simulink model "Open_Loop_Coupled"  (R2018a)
settings: Solver=ode45  StartTime=0.0  StopTime=80  RelTol=1e-3  EnableMultiTasking=on
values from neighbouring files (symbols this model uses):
  Aact = [0, 1; -omg^2, -2*zet*omg]    [init.m]
  Bact = [0; omg^2]    [init.m]
  Cact = [1, 0]    [init.m]
  Cyb = -0.0245    [init.m]    (also in lqr_des.m)
  Cydel = [-0.24668,0.24668, 0.47413,-0.47413,0]/100    [init.m]    (also in lqr_des.m = [-0.24668,0.24668, 0.47413,-0.47413]/100)
  Cza = -0.073    [init.m]
  Czdel = [0.51664,0.51664,0.60478,0.60478,0.06]/100    [init.m]
  d2r = pi/180    (= 0.0174532925199)    [init.m]
  Dact = 0    [init.m]
  Mass = 198.32    [init.m]    (also in lqr_des.m)
  Qbar = 150    [init.m]    (also in lqr_des.m)
  r2d = 180/pi    (= 57.2957795131)    [init.m]    (also in pl.m)
  Sref = 79.069    [init.m]    (also in lqr_des.m)
  V0 = 822.8    [init.m]
undefined symbols (not defined in the file or in its folder): Ap, Bp, Cp, Dp, K4axmix, Kpr, Kq

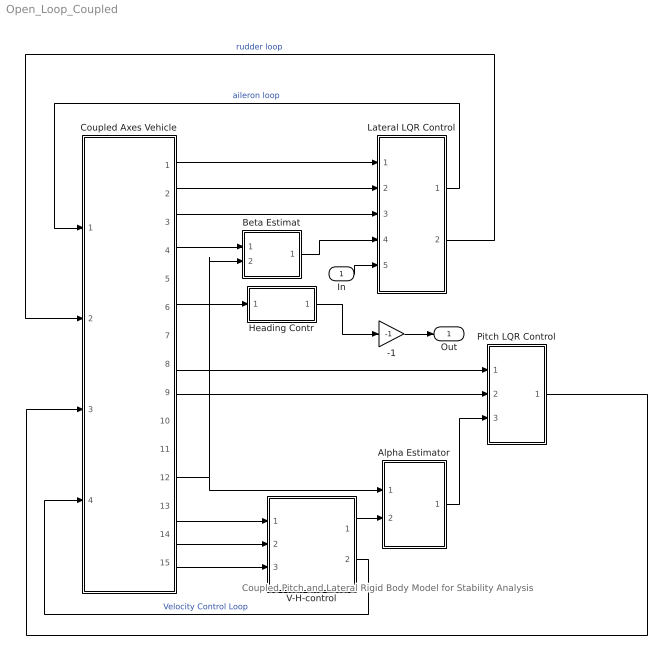
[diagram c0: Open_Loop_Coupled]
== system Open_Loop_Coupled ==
  note: Coupled Pitch and Lateral Rigid Body Model for Stability Analysis
  In : Inport
  -1 : Gain  Gain=-1
  Alpha Estimator : Subsystem
  Beta Estimat : Subsystem
  Coupled Axes Vehicle : Subsystem
  Heading Contr : Subsystem
  Lateral LQR Control : Subsystem
  Pitch LQR Control : Subsystem
  V-H-control : Subsystem
  Out : Outport
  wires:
  Coupled Axes Vehicle/2(p) -> Lateral LQR Control/2(p)
  Coupled Axes Vehicle/3(r) -> Lateral LQR Control/3(r)
  Coupled Axes Vehicle/1(phi) -> Lateral LQR Control/1(phi)
  Coupled Axes Vehicle/9(q) -> Pitch LQR Control/2(q)
  Coupled Axes Vehicle/8(thet) -> Pitch LQR Control/1(thet)
  Coupled Axes Vehicle/12(delt) -> Alpha Estimator/1(delta), Beta Estimat/2(delta)
  Alpha Estimator/1(alphat) -> Pitch LQR Control/3(alfa)
  V-H-control/1(Zdd-com) -> Alpha Estimator/2(Zdd)
  V-H-control/2(Throtle) -> Coupled Axes Vehicle/4(Ax-cmd)  "Velocity Control Loop"
  Coupled Axes Vehicle/4(Ny) -> Beta Estimat/1(Ydd)
  Beta Estimat/1(bethat) -> Lateral LQR Control/4(bet)
  Coupled Axes Vehicle/6("chi ") -> Heading Contr/1(chi)
  Coupled Axes Vehicle/14(Nz) -> V-H-control/2(Az)
  Coupled Axes Vehicle/15(dH) -> V-H-control/3(dH)
  Coupled Axes Vehicle/13(V-dot) -> V-H-control/1(Vdot)
  -1/1 -> Out/1
  Lateral LQR Control/2(Rud) -> Coupled Axes Vehicle/2(yaw)  "rudder loop"
  Lateral LQR Control/1(Ailer) -> Coupled Axes Vehicle/1(roll)  "aileron loop"
  Heading Contr/1(phi-cmd) -> -1/1
  In/1 -> Lateral LQR Control/5(ph-cmd)
  Pitch LQR Control/1(elev) -> Coupled Axes Vehicle/3(pitch)

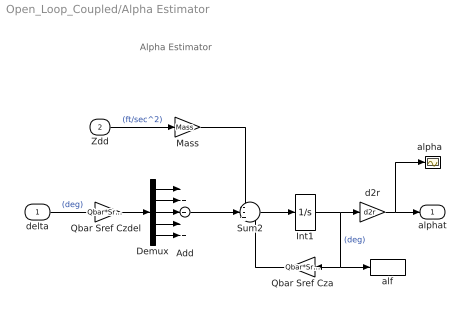
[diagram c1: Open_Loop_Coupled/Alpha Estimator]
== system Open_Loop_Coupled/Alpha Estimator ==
  note: Alpha Estimator
  delta : Inport
  Zdd : Inport  Port=2
  Add : Sum  Inputs=+++++
  Demux : Demux  Outputs=5
  Int1 : Integrator
  Mass : Gain  Gain=Mass
  Qbar Sref Cza : Gain  Gain=Qbar*Sref*Cza
  "Qbar Sref Czdel " : Gain  Gain=Qbar*Sref*Czdel
  Sum2 : Sum  Inputs=--+
  alf : ToWorkspace  VariableName=alphat  SampleTime=-1
  "alpha  " : Scope
  d2r : Gain  Gain=d2r
  alphat : Outport
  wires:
  Demux/5 -> Add/5
  Demux/4 -> Add/4
  Demux/3 -> Add/3
  Demux/2 -> Add/2
  Demux/1 -> Add/1
  "Qbar Sref Czdel "/1 -> Demux/1
  delta/1 -> "Qbar Sref Czdel "/1  "(deg)"
  Sum2/1 -> Int1/1
  Int1/1 -> d2r/1, Qbar Sref Cza/1, alf/1  "(deg)"
  Qbar Sref Cza/1 -> Sum2/3
  Zdd/1 -> Mass/1  "(ft/sec^2)"
  Mass/1 -> Sum2/1
  d2r/1 -> "alpha  "/1, alphat/1
  Add/1 -> Sum2/2

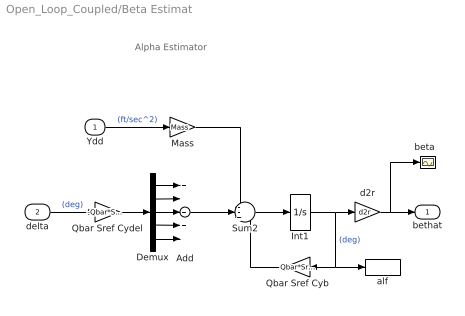
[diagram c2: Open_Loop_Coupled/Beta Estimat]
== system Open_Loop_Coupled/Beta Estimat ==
  note: Alpha Estimator
  Ydd : Inport
  delta : Inport  Port=2
  Add : Sum  Inputs=+++++
  Demux : Demux  Outputs=5
  Int1 : Integrator
  Mass : Gain  Gain=Mass
  Qbar Sref Cyb : Gain  Gain=Qbar*Sref*Cyb
  Qbar Sref Cydel : Gain  Gain=-Qbar*Sref*Cydel
  Sum2 : Sum  Inputs=--+
  alf : ToWorkspace  VariableName=bethat  SampleTime=-1
  "beta  " : Scope
  d2r : Gain  Gain=d2r
  bethat : Outport
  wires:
  Add/1 -> Sum2/2
  d2r/1 -> bethat/1, "beta  "/1
  Mass/1 -> Sum2/1
  Ydd/1 -> Mass/1  "(ft/sec^2)"
  Qbar Sref Cyb/1 -> Sum2/3
  Int1/1 -> alf/1, Qbar Sref Cyb/1, d2r/1  "(deg)"
  Sum2/1 -> Int1/1
  delta/1 -> Qbar Sref Cydel/1  "(deg)"
  Qbar Sref Cydel/1 -> Demux/1
  Demux/1 -> Add/1
  Demux/2 -> Add/2
  Demux/3 -> Add/3
  Demux/4 -> Add/4
  Demux/5 -> Add/5

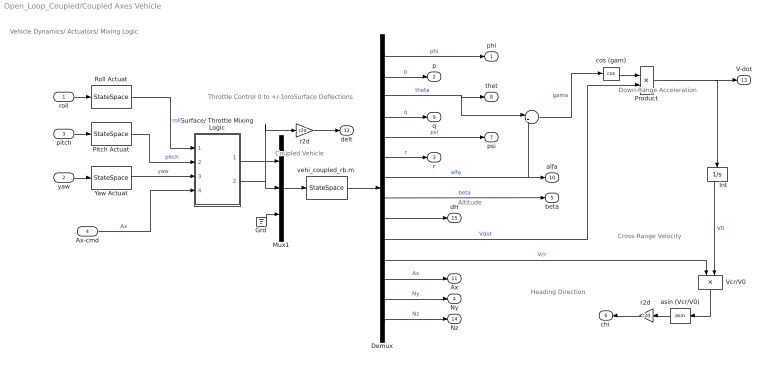
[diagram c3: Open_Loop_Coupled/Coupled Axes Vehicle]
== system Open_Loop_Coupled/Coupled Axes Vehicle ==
  note: Altitude
  note: Cross-Range Velocity
  note: Coupled Vehicle
  note: AeroSurface Deflections
  note: Vehicle Dynamics/ Actuators/ Mixing Logic
  note: Heading Direction
  note: Down-Range Acceleration
  note: Throttle Control 0 to +/-1
  roll : Inport
  yaw : Inport  Port=2
  pitch : Inport  Port=3
  Ax-cmd : Inport  Port=4
  "    " : Sum  Inputs=|+-
  Demux : Demux  Outputs=14
  Grd : Ground
  Int : Integrator  InitialCondition=V0
  Mux1 : Mux  Inputs=[1, 5, 1]
  Pitch Actuat : StateSpace  A=Aact  B=Bact  C=Cact  D=Dact  InitialCondition=0
  Product : Product
  Roll Actuat : StateSpace  A=Aact  B=Bact  C=Cact  D=Dact  InitialCondition=0
  Surface/ Throttle Mixing Logic : Subsystem
  Vcr/V0 : Product  Inputs=*/
  Yaw Actuat : StateSpace  A=Aact  B=Bact  C=Cact  D=Dact  InitialCondition=0
  asin (Vcr/V0) : Trigonometry  Operator=asin
  cos (gam) : Trigonometry  Operator=cos
  r2d : Gain  Gain=r2d
  "r2d " : Gain  Gain=r2d
  "vehi_coupled_rb.m " : StateSpace  A=Ap  B=Bp  C=Cp  D=Dp  InitialCondition=0
  phi : Outport
  p : Outport  Port=2
  r : Outport  Port=3
  Ny : Outport  Port=4
  beta : Outport  Port=5
  "chi " : Outport  Port=6
  psi : Outport  Port=7
  thet : Outport  Port=8
  q : Outport  Port=9
  alfa : Outport  Port=10
  Ax : Outport  Port=11
  delt : Outport  Port=12
  V-dot : Outport  Port=13
  Nz : Outport  Port=14
  dH : Outport  Port=15
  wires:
  asin (Vcr/V0)/1 -> "r2d "/1
  Vcr/V0/1 -> asin (Vcr/V0)/1
  "r2d "/1 -> "chi "/1
  Int/1 -> Vcr/V0/2  "V0"
  Demux/10 -> Product/2  "Vdot"
  Product/1 -> V-dot/1, Int/1
  cos (gam)/1 -> Product/1
  "    "/1 -> cos (gam)/1  "gama"
  Surface/ Throttle Mixing Logic/2(delta) -> r2d/1, Mux1/2
  Surface/ Throttle Mixing Logic/1(Thro) -> Mux1/1
  r2d/1 -> delt/1
  Demux/14 -> Nz/1  "Nz"
  Demux/13 -> Ny/1  "Ny"
  Demux/12 -> Ax/1  "Ax"
  Demux/11 -> Vcr/V0/1  "Vcr"
  Demux/9 -> dH/1
  Demux/8 -> beta/1  "beta"
  Demux/7 -> "    "/2, alfa/1  "alfa"
  Demux/6 -> r/1  "r"
  Demux/5 -> psi/1  "psi"
  Demux/4 -> q/1  "q"
  Demux/3 -> "    "/1, thet/1  "theta"
  "vehi_coupled_rb.m "/1 -> Demux/1
  Ax-cmd/1 -> Surface/ Throttle Mixing Logic/4(Ax)  "Ax"
  Pitch Actuat/1 -> Surface/ Throttle Mixing Logic/2(ptch)  "pitch"
  Roll Actuat/1 -> Surface/ Throttle Mixing Logic/1(roll)  "roll"
  pitch/1 -> Pitch Actuat/1
  yaw/1 -> Yaw Actuat/1
  roll/1 -> Roll Actuat/1
  Demux/2 -> p/1  "p"
  Demux/1 -> phi/1  "phi"
  Yaw Actuat/1 -> Surface/ Throttle Mixing Logic/3(yaw)  "yaw"
  Mux1/1 -> "vehi_coupled_rb.m "/1
  Grd/1 -> Mux1/3

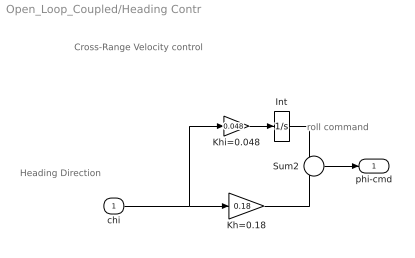
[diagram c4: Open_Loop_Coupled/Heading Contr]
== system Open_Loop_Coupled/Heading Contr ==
  note: Cross-Range Velocity control
  note: Heading Direction
  note: roll command
  chi : Inport
  Int : Integrator
  Kh=0.18 : Gain  Gain=0.18
  Khi=0.048 : Gain  Gain=0.048
  Sum2 : Sum  Inputs=--
  phi-cmd : Outport
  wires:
  Khi=0.048/1 -> Int/1
  Kh=0.18/1 -> Sum2/2
  Int/1 -> Sum2/1
  Sum2/1 -> phi-cmd/1
  chi/1 -> Kh=0.18/1, Khi=0.048/1

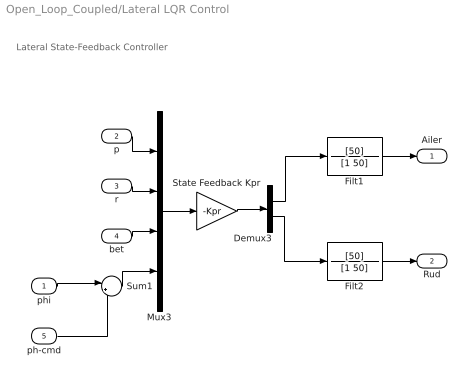
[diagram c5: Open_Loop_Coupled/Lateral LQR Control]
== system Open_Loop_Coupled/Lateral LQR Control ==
  note: Lateral State-Feedback Controller
  phi : Inport
  p : Inport  Port=2
  r : Inport  Port=3
  bet : Inport  Port=4
  ph-cmd : Inport  Port=5
  Demux3 : Demux  Outputs=2
  Filt1 : TransferFcn  Numerator=[50]  Denominator=[1 50]
  Filt2 : TransferFcn  Numerator=[50]  Denominator=[1 50]
  Mux3 : Mux
  State Feedback Kpr : Gain  Gain=-Kpr  Multiplication=Matrix(K*u) (u vector)
  Sum1 : Sum  Inputs=|+-
  Ailer : Outport
  Rud : Outport  Port=2
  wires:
  State Feedback Kpr/1 -> Demux3/1
  ph-cmd/1 -> Sum1/2
  phi/1 -> Sum1/1
  Sum1/1 -> Mux3/4
  Filt1/1 -> Ailer/1
  Filt2/1 -> Rud/1
  Demux3/2 -> Filt2/1
  Demux3/1 -> Filt1/1
  bet/1 -> Mux3/3
  r/1 -> Mux3/2
  p/1 -> Mux3/1
  Mux3/1 -> State Feedback Kpr/1

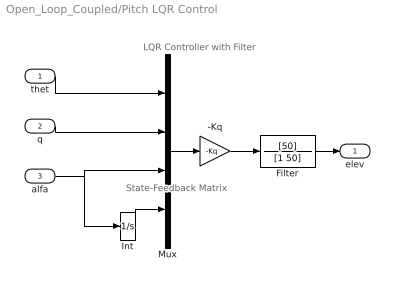
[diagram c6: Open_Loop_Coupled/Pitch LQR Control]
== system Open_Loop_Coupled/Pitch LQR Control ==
  note: State-Feedback Matrix
  note: LQR Controller with Filter
  thet : Inport
  q : Inport  Port=2
  alfa : Inport  Port=3
  -Kq : Gain  Gain=-Kq  Multiplication=Matrix(K*u)
  Filter : TransferFcn  Numerator=[50]  Denominator=[1 50]
  Int : Integrator
  Mux : Mux
  elev : Outport
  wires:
  alfa/1 -> Int/1, Mux/3
  thet/1 -> Mux/1
  q/1 -> Mux/2
  Filter/1 -> elev/1
  Int/1 -> Mux/4
  Mux/1 -> -Kq/1
  -Kq/1 -> Filter/1

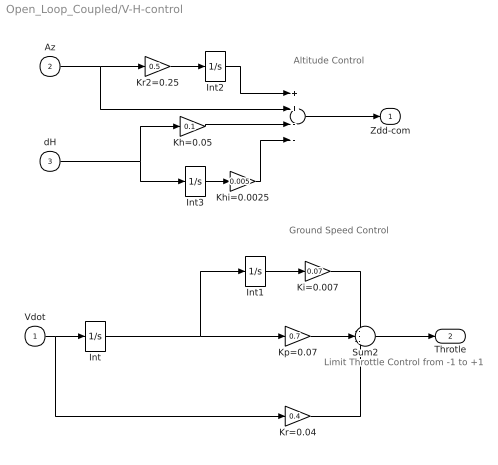
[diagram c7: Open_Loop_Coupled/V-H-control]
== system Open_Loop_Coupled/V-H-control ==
  note: Altitude Control
  note: Ground Speed Control
  note: Limit Throttle Control from -1 to +1
  Vdot : Inport
  Az : Inport  Port=2
  dH : Inport  Port=3
  "  " : Sum  Inputs=++--
  Int{,1..3} (4 alike) : Integrator
  Kh=0.05 : Gain  Gain=0.1
  Khi=0.0025 : Gain  Gain=0.005
  Ki=0.007 : Gain  Gain=0.07
  Kp=0.07 : Gain  Gain=0.7
  Kr2=0.25 : Gain  Gain=0.5
  Kr=0.04 : Gain  Gain=0.4
  Sum2 : Sum  Inputs=---
  Zdd-com : Outport
  Throtle : Outport  Port=2
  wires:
  Khi=0.0025/1 -> "  "/4
  Int3/1 -> Khi=0.0025/1
  "  "/1 -> Zdd-com/1
  Az/1 -> "  "/2, Kr2=0.25/1
  Int2/1 -> "  "/1
  Kr2=0.25/1 -> Int2/1
  Kh=0.05/1 -> "  "/3
  dH/1 -> Int3/1, Kh=0.05/1
  Int/1 -> Int1/1, Kp=0.07/1
  Int1/1 -> Ki=0.007/1
  Ki=0.007/1 -> Sum2/1
  Kp=0.07/1 -> Sum2/2
  Kr=0.04/1 -> Sum2/3
  Sum2/1 -> Throtle/1
  Vdot/1 -> Kr=0.04/1, Int/1

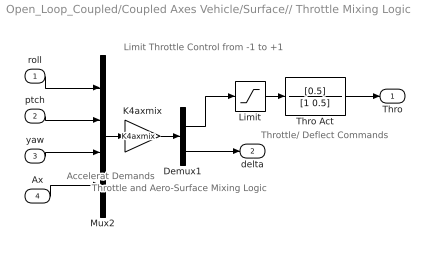
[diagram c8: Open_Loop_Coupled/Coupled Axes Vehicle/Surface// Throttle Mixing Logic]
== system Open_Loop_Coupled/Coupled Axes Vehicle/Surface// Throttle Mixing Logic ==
  note: Throttle/ Deflect Commands
  note: Accelerat Demands
  note: Throttle and Aero-Surface Mixing Logic
  note: Limit Throttle Control from -1 to +1
  roll : Inport
  ptch : Inport  Port=2
  yaw : Inport  Port=3
  Ax : Inport  Port=4
  Demux1 : Demux  Outputs=[1, 5]
  K4axmix : Gain  Gain=K4axmix  Multiplication=Matrix(K*u) (u vector)
  Limit : Saturate  UpperLimit=1  LowerLimit=-1
  Mux2 : Mux
  Thro Act : TransferFcn  Numerator=[0.5]  Denominator=[1 0.5]
  Thro : Outport
  delta : Outport  Port=2
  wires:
  ptch/1 -> Mux2/2
  yaw/1 -> Mux2/3
  Ax/1 -> Mux2/4
  roll/1 -> Mux2/1
  Demux1/2 -> delta/1
  Demux1/1 -> Limit/1
  Mux2/1 -> K4axmix/1
  K4axmix/1 -> Demux1/1
  Limit/1 -> Thro Act/1
  Thro Act/1 -> Thro/1
